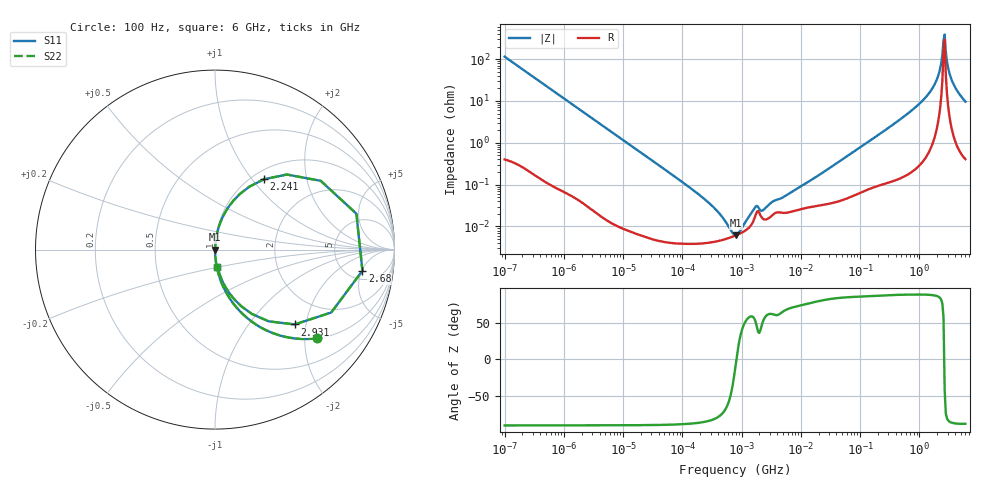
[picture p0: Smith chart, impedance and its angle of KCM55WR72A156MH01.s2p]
!Murata Part Number: KCM55WR72A156MH01
!These Parameters are Measured in Series Mode Connection
!Data Generated on Mar 13, 2026
!  o--ll--o
!Port1  Port2
!  o------o
!Operation Temp=25[degC], DC Bias Voltage=0[V]
!Freq. Start=100[Hz] Stop=6[GHz] 401[Steps]
# Hz S RI R 50
!Freq.(Hz) S11(Real) S11(Imag) S21(Real) S21(Imag) S12(Real) S12(Imag) S22(Real) S22(Imag)
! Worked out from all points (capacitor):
!   401 points, 100 Hz to 6 GHz, reference 50 ohm
!   read as one part in series: C = 13.9 uF near 109 Hz
!   lowest |Z| = 6.19 mohm at 810.1 kHz (marker M1)
!   series resonance near 817.9 kHz, so ESL is about 2.7 nH
!   S11 on the Smith chart (normalised r, x): 100 Hz: 1.01, -2.29; 2.241 GHz: 1.13, +1.15; 2.68 GHz: 6.81, -5.14; 2.931 GHz: 1.30, -1.73; 6 GHz: 1.01, -0.19
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100  0.5675 -0.4937  0.4325 0.4937  0.4325 0.4937  0.5675 -0.4937
350  0.0985 -0.2957  0.9015 0.2957  0.9015 0.2957  0.0985 -0.2957
2008  0.00368 -0.0574  0.9963 0.0574  0.9963 0.0574  0.00368 -0.0574
40335  5.35e-05 -0.00289  0.9999 0.00289  0.9999 0.00289  5.35e-05 -0.00289
252896  4.04e-05 -0.000415  1 0.000415  1 0.000415  4.04e-05 -0.000415
592111  5.23e-05 -9.12e-05  0.9999 9.12e-05  0.9999 9.12e-05  5.23e-05 -9.12e-05
774597  6.02e-05 -1.5e-05  0.9999 1.5e-05  0.9999 1.5e-05  6.02e-05 -1.5e-05
810067  6.18e-05 -2.6e-06  0.9999 2.6e-06  0.9999 2.6e-06  6.18e-05 -2.6e-06
1059725  7.41e-05 7.25e-05  0.9999 -7.25e-05  0.9999 -7.25e-05  7.41e-05 7.25e-05
1734173  0.000192 0.00023  0.9998 -0.00023  0.9998 -0.00023  0.000192 0.00023
2268635  0.000154 0.000186  0.9998 -0.000186  0.9998 -0.000186  0.000154 0.000186
1.555665e7  0.000298 0.0013  0.9997 -0.0013  0.9997 -0.0013  0.000298 0.0013
3.124326e8  0.00168 0.0235  0.9983 -0.0235  0.9983 -0.0235  0.00168 0.0235
1.251881e9  0.0177 0.1151  0.9823 -0.1151  0.9823 -0.1151  0.0177 0.1151
1.873145e9  0.0818 0.2465  0.9182 -0.2465  0.9182 -0.2465  0.0818 0.2465
2.240541e9  0.272 0.3916  0.728 -0.3916  0.728 -0.3916  0.272 0.3916
2.450438e9  0.5894 0.3831  0.4106 -0.3831  0.4106 -0.3831  0.5894 0.3831
2.679998e9  0.8214 -0.1176  0.1786 0.1176  0.1786 0.1176  0.8214 -0.1176
2.931063e9  0.4437 -0.417  0.5563 0.417  0.5563 0.417  0.4437 -0.417
3.205649e9  0.2062 -0.3587  0.7938 0.3587  0.7938 0.3587  0.2062 -0.3587
3.666503e9  0.0845 -0.2487  0.9155 0.2487  0.9155 0.2487  0.0845 -0.2487
6e9  0.0131 -0.0944  0.9869 0.0944  0.9869 0.0944  0.0131 -0.0944
